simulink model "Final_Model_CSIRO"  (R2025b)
settings: Solver=ode23tb  StartTime=0.0  StopTime=50  RelTol=1e-3
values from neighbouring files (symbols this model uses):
  C_4 = 0.1670*C_b    (= 1.00487241952e-06)    [VSM_CSIRO.m]    (also in VSM.m)
  C_6 = 0.2835*C_b    (= 1.70587623314e-06)    [VSM_CSIRO.m]    (also in VSM.m)
  C_8 = 0.2275*C_b    (= 1.36891302659e-06)    [VSM_CSIRO.m]    (also in VSM.m)
  C_dc = 0.008*(n)    (= 1.6)    [VSM_CSIRO.m]    (also in VSM.m)
  C_f = n*300*10^-6    (= 0.06)    [VSM_CSIRO.m]    (also in VSM.m)
  D_p = (1/(m_p*w_b))    (= 101321.183642)    [VSM_CSIRO.m]    (also in VSM.m)
  droop_percentage = 1    [VSM_CSIRO.m]    (also in VSM.m = 5)
  i_ll = -1.15*(S_b/Vdc_n)-i_loss_dc    [VSM_CSIRO.m]    (also in VSM.m)
  i_ul = 1.15*(S_b/Vdc_n)+i_loss_dc    [VSM_CSIRO.m]    (also in VSM.m)
  J = D_p*tau_f    (= 2026.42367285)    [VSM_CSIRO.m]    (also in VSM.m)
  k_dc = eta_1/(Vdc_n*m_p)    [VSM_CSIRO.m]    (also in VSM.m)
  K_p = (1/Vdc_n)    [VSM_CSIRO.m]    (also in VSM.m)
  K_r = 1/R_dc    [VSM_CSIRO.m]    (also in VSM.m)
  Kff_i = 1    [VSM_CSIRO.m]    (also in VSM.m)
  Kff_v = 1    [VSM_CSIRO.m]    (also in VSM.m)
  Ki_i = (1/n)*1.19    (= 0.00595)    [VSM_CSIRO.m]    (also in VSM.m)
  Ki_v = (n)*1.161022    (= 232.2044)    [VSM_CSIRO.m]    (also in VSM.m)
  ki_v_ac = 4*5.2500e-04    (= 0.0021)    [VSM_CSIRO.m]    (also in VSM.m)
  Kp_i = 0.738891    [VSM_CSIRO.m]    (also in VSM.m)
  Kp_v = 0.52    [VSM_CSIRO.m]    (also in VSM.m)
  kp_v_ac = 0.001    [VSM_CSIRO.m]    (also in VSM.m)
  L1_pu = 1*0.0186/m    (= 0.000186)    [VSM_CSIRO.m]    (also in VSM.m)
  L_45 = L_lines(2)    [VSM_CSIRO.m]    (also in VSM.m)
  L_56 = L_lines(3)    [VSM_CSIRO.m]    (also in VSM.m)
  L_67 = L_lines(5)    [VSM_CSIRO.m]    (also in VSM.m)
  L_78 = L_lines(6)    [VSM_CSIRO.m]    (also in VSM.m)
  L_89 = L_lines(8)    [VSM_CSIRO.m]    (also in VSM.m)
  L_94 = L_lines(9)    [VSM_CSIRO.m]    (also in VSM.m)
  L_f = (1/n)*200*10^-6    (= 1e-06)    [VSM_CSIRO.m]    (also in VSM.m)
  n = 200    [VSM_CSIRO.m]    (also in VSM.m)
  pl = S_b*ps    (= 75000000)    [VSM_CSIRO.m]    (also in VSM.m)
  ps = base/3    (= 0.75)    [VSM_CSIRO.m]    (also in VSM.m)
  R1_pu = 1*0.00734/m    (= 7.34e-05)    [VSM_CSIRO.m]    (also in VSM.m)
  R_45 = R_lines(2)    [VSM_CSIRO.m]    (also in VSM.m)
  R_56 = R_lines(3)    [VSM_CSIRO.m]    (also in VSM.m)
  R_67 = R_lines(5)    [VSM_CSIRO.m]    (also in VSM.m)
  R_78 = R_lines(6)    [VSM_CSIRO.m]    (also in VSM.m)
  R_89 = R_lines(8)    [VSM_CSIRO.m]    (also in VSM.m)
  R_94 = R_lines(9)    [VSM_CSIRO.m]    (also in VSM.m)
  R_dc = (Vdc_n/(0.05*(S_b)/Vdc_n))    [VSM_CSIRO.m]    (also in VSM.m)
  R_f = 0.001/n    (= 5e-06)    [VSM_CSIRO.m]    (also in VSM.m)
  S_b = 100*(10^6)    (= 100000000)    [VSM_CSIRO.m]    (also in VSM.m)
  S_bt = S_b    (= 100000000)    [VSM_CSIRO.m]    (also in VSM.m)
  T_en = T_load-0.5    (= 44.5)    [VSM_CSIRO.m]    (also in VSM.m = 24.5)
  t_l = 2    [VSM_CSIRO.m]
  tau_dc = 0.05    [VSM_CSIRO.m]    (also in VSM.m)
  tau_g = 5    [VSM_CSIRO.m]    (also in VSM.m)
  V1_rms = 1000    [VSM_CSIRO.m]    (also in VSM.m)
  V2_rms = 13800    [VSM_CSIRO.m]    (also in VSM.m)
  V_m = sqrt(2/3)*V1_rms    [VSM_CSIRO.m]    (also in VSM.m)
  Vdc_n = 3*V_m    [VSM_CSIRO.m]    (also in VSM.m)
  w_b = 2*pi*f_b    (= 314.159265359)    [VSM_CSIRO.m]    (also in VSM.m)
  w_f = 2*pi*5    (= 31.4159265359)    [VSM_CSIRO.m]    (also in VSM.m)
undefined symbols (not defined in the file or in its folder): D1, Delta, DiscIntNeverNeededParam, i_dc
libraries: spsSeriesRLCBranchLib x142, spsThreePhaseVIMeasurementLib x69, slpidlib x44, spsabctodq0Lib x44, spsVoltageMeasurementLib x28, spsGroundLib x23, spsThreePhaseBreakerLib x23, spsThreePhaseParallelRLCLoadLib x21, spsdq0toabcLib x16, spsUniversalBridgeLib x16, spsPowerPositiveSequenceLib x14, spsDCVoltageSourceLib x14
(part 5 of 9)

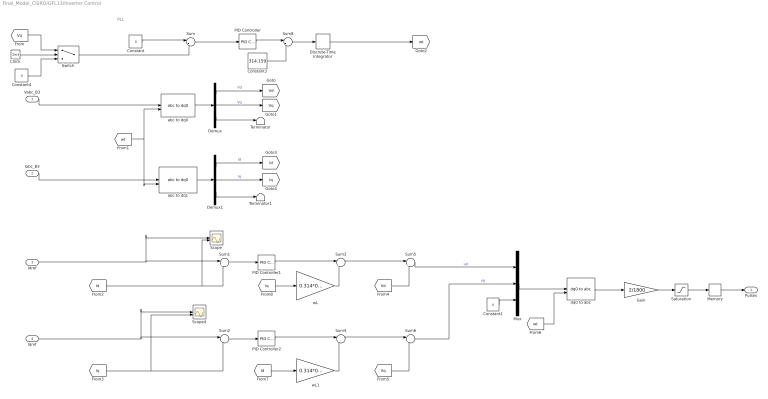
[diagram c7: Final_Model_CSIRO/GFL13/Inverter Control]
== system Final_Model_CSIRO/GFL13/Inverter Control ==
  note: PLL
  Vabc_B3 : Inport
  Iabc_B3 : Inport  Port=2
  Idref : Inport  Port=3
  Iqref : Inport  Port=4
  Clock : Clock
  Constant : Constant  Value=0  SampleTime=-1
  Constant1 : Constant  Value=0  SampleTime=-1
  Constant3 : Constant  Value=314.159  SampleTime=-1
  Constant4 : Constant  Value=0
  Demux : Demux  Outputs=3
  Demux1 : Demux  Outputs=3
  Discrete-Time Integrator : DiscreteIntegrator  SampleTime=-1  ICPrevOutput=DiscIntNeverNeededParam  ICPrevScaledInput=DiscIntNeverNeededParam
  Gain : Gain  Gain=2/1800
  Memory : Memory
  Mux : Mux  Inputs=3
  PID Controller : slpidlib/PID Controller  Controller=PI  Form=Parallel  TimeDomain=Discrete-time  UseExternalTs=off  SampleTime=-1  IntegratorMethod=Forward Euler  FilterMethod=Forward Euler  ControllerParametersSource=internal  P=0.02  I=50  UseKiTs=off  D=0  UseExternalDerivativeSource=off  N=100  UseFilter=on  TunerSelectOption=Transfer Function Based (PID Tuner App)  InitialConditionSource=internal  InitialConditionForIntegrator=0  InitialConditionForFilter=0  DifferentiatorICPrevScaledInput=0  ExternalReset=none  TrackingMode=off  Kt=1  LimitOutput=off  SatLimitsSource=internal  UpperSaturationLimit=inf  LowerSaturationLimit=-inf  LinearizeAsGain=on  AntiWindupMode=none  Kb=1  LimitIntegrator=off  UpperIntegratorSaturationLimit=inf  LowerIntegratorSaturationLimit=-inf  POutMin=[]  POutMax=[]  IOutMin=[]  IOutMax=[]  DOutMin=[]  DOutMax=[]  NOutMin=[]  NOutMax=[]  SumOutMin=[]  SumOutMax=[]  SaturationOutMin=[]  SaturationOutMax=[]  PParamMin=[]  PParamMax=[]  IParamMin=[]  IParamMax=[]  DParamMin=[]  DParamMax=[]  NParamMin=[]  NParamMax=[]  KbParamMin=[]  KbParamMax=[]  KtParamMin=[]  KtParamMax=[]  KbOutMin=[]  KbOutMax=[]  KtOutMin=[]  KtOutMax=[]  IntegratorOutMin=[]  IntegratorOutMax=[]  FilterOutMin=[]  FilterOutMax=[]  SumI1OutMin=[]  SumI1OutMax=[]  SumI2OutMin=[]  SumI2OutMax=[]  SumI3OutMin=[]  SumI3OutMax=[]  SumI4OutMin=[]  SumI4OutMax=[]  SumDOutMin=[]  SumDOutMax=[]  DifferentiatorOutMin=[]  DifferentiatorOutMax=[]  FilterDiffOutCoefMin=[]  FilterDiffOutCoefMax=[]  ReciprocalOutMin=[]  ReciprocalOutMax=[]  SumDenOutMin=[]  SumDenOutMax=[]  SumNumOutMin=[]  SumNumOutMax=[]  DivideOutMin=[]  DivideOutMax=[]  UdiffTsProdOutMin=[]  UdiffTsProdOutMax=[]  NTsProdOutMin=[]  NTsProdOutMax=[]  UintegralTsProdOutMin=[]  UintegralTsProdOutMax=[]  UngainTsProdOutMin=[]  UngainTsProdOutMax=[]  ClampingZeroOutDataTypeStr=Inherit: Inherit via back propagation  ClampingZeroOutMin=[]  ClampingZeroOutMax=[]  FilterDenConstantOutDataTypeStr=Inherit: Inherit via back propagation  FilterDenConstantOutMin=[]  FilterDenConstantOutMax=[]  PCopyOutDataTypeStr=Inherit: Inherit via back propagation  PCopyOutMin=[]  PCopyOutMax=[]  NCopyOutDataTypeStr=Inherit: Inherit via back propagation  NCopyOutMin=[]  NCopyOutMax=[]  IntegratorContinuousStateAttributes=''  IntegratorStateMustResolveToSignalObject=off  IntegratorRTWStateStorageClass=Auto  FilterContinuousStateAttributes=''  FilterStateMustResolveToSignalObject=off  FilterRTWStateStorageClass=Auto  ParallelPVariant=InternalParameters  IdealPVariant=Disabled  IVariant=InternalParameters  DVariant=Disabled  IntegratorVariant=Discrete  SatVariant=Disabled  AWVariant=Passthrough  PCopyVariant=Disabled  TRVariant=Disabled  FdbkBlocksVariant=Forward  IdealPFdbkVariant=Disabled  SatFdbkVariant=Disabled  DerivativeFilterVariant=Disabled  NVariant=Disabled  NCopyVariant=Disabled_SignalSpec  FilterICVariant=Disabled  IntegratorICVariant=InternalICs  ExternalResetVariant=Disabled  TRSumVariant=Passthrough  SumFdbkVariant=Disabled  SumVariant=Sum_PI  TsampFilterVariant=InternalTs  TsampNgainVariant=Passthrough  TsampIntegralVariant=Disabled_SignalSpec  ExternalSaturationOutDataTypeStr=Inherit: Same as second input  DerivativeSourceVariant=Disabled  PreIntVariant=InternalPreInt
  PID Controller1 : slpidlib/PID Controller  Controller=PI  Form=Parallel  TimeDomain=Discrete-time  UseExternalTs=off  SampleTime=-1  IntegratorMethod=Forward Euler  FilterMethod=Forward Euler  ControllerParametersSource=internal  P=0.1  I=10000/200  UseKiTs=off  D=0  UseExternalDerivativeSource=off  N=100  UseFilter=on  TunerSelectOption=Transfer Function Based (PID Tuner App)  InitialConditionSource=internal  InitialConditionForIntegrator=0  InitialConditionForFilter=0  DifferentiatorICPrevScaledInput=0  ExternalReset=none  TrackingMode=off  Kt=1  LimitOutput=on  SatLimitsSource=internal  UpperSaturationLimit=20e3  LowerSaturationLimit=-20e3  LinearizeAsGain=on  AntiWindupMode=none  Kb=1  LimitIntegrator=off  UpperIntegratorSaturationLimit=inf  LowerIntegratorSaturationLimit=-inf  POutMin=[]  POutMax=[]  IOutMin=[]  IOutMax=[]  DOutMin=[]  DOutMax=[]  NOutMin=[]  NOutMax=[]  SumOutMin=[]  SumOutMax=[]  SaturationOutMin=[]  SaturationOutMax=[]  PParamMin=[]  PParamMax=[]  IParamMin=[]  IParamMax=[]  DParamMin=[]  DParamMax=[]  NParamMin=[]  NParamMax=[]  KbParamMin=[]  KbParamMax=[]  KtParamMin=[]  KtParamMax=[]  KbOutMin=[]  KbOutMax=[]  KtOutMin=[]  KtOutMax=[]  IntegratorOutMin=[]  IntegratorOutMax=[]  FilterOutMin=[]  FilterOutMax=[]  SumI1OutMin=[]  SumI1OutMax=[]  SumI2OutMin=[]  SumI2OutMax=[]  SumI3OutMin=[]  SumI3OutMax=[]  SumI4OutMin=[]  SumI4OutMax=[]  SumDOutMin=[]  SumDOutMax=[]  DifferentiatorOutMin=[]  DifferentiatorOutMax=[]  FilterDiffOutCoefMin=[]  FilterDiffOutCoefMax=[]  ReciprocalOutMin=[]  ReciprocalOutMax=[]  SumDenOutMin=[]  SumDenOutMax=[]  SumNumOutMin=[]  SumNumOutMax=[]  DivideOutMin=[]  DivideOutMax=[]  UdiffTsProdOutMin=[]  UdiffTsProdOutMax=[]  NTsProdOutMin=[]  NTsProdOutMax=[]  UintegralTsProdOutMin=[]  UintegralTsProdOutMax=[]  UngainTsProdOutMin=[]  UngainTsProdOutMax=[]  ClampingZeroOutDataTypeStr=Inherit: Inherit via back propagation  ClampingZeroOutMin=[]  ClampingZeroOutMax=[]  FilterDenConstantOutDataTypeStr=Inherit: Inherit via back propagation  FilterDenConstantOutMin=[]  FilterDenConstantOutMax=[]  PCopyOutDataTypeStr=Inherit: Inherit via back propagation  PCopyOutMin=[]  PCopyOutMax=[]  NCopyOutDataTypeStr=Inherit: Inherit via back propagation  NCopyOutMin=[]  NCopyOutMax=[]  IntegratorContinuousStateAttributes=''  IntegratorStateMustResolveToSignalObject=off  IntegratorRTWStateStorageClass=Auto  FilterContinuousStateAttributes=''  FilterStateMustResolveToSignalObject=off  FilterRTWStateStorageClass=Auto  ParallelPVariant=InternalParameters  IdealPVariant=Disabled  IVariant=InternalParameters  DVariant=Disabled  IntegratorVariant=Discrete  SatVariant=Enabled  AWVariant=Passthrough  PCopyVariant=Disabled  TRVariant=Disabled  FdbkBlocksVariant=Forward  IdealPFdbkVariant=Disabled  SatFdbkVariant=Disabled  DerivativeFilterVariant=Disabled  NVariant=Disabled  NCopyVariant=Disabled_SignalSpec  FilterICVariant=Disabled  IntegratorICVariant=InternalICs  ExternalResetVariant=Disabled  TRSumVariant=Passthrough  SumFdbkVariant=Disabled  SumVariant=Sum_PI  TsampFilterVariant=InternalTs  TsampNgainVariant=Passthrough  TsampIntegralVariant=Disabled_SignalSpec  ExternalSaturationOutDataTypeStr=Inherit: Same as second input  DerivativeSourceVariant=Disabled  PreIntVariant=InternalPreInt
  PID Controller2 : slpidlib/PID Controller  Controller=PI  Form=Parallel  TimeDomain=Discrete-time  UseExternalTs=off  SampleTime=-1  IntegratorMethod=Forward Euler  FilterMethod=Forward Euler  ControllerParametersSource=internal  P=0.1  I=1000/2  UseKiTs=off  D=0  UseExternalDerivativeSource=off  N=100  UseFilter=on  TunerSelectOption=Transfer Function Based (PID Tuner App)  InitialConditionSource=internal  InitialConditionForIntegrator=0  InitialConditionForFilter=0  DifferentiatorICPrevScaledInput=0  ExternalReset=none  TrackingMode=off  Kt=1  LimitOutput=on  SatLimitsSource=internal  UpperSaturationLimit=20e3  LowerSaturationLimit=-20e3  LinearizeAsGain=on  AntiWindupMode=none  Kb=1  LimitIntegrator=off  UpperIntegratorSaturationLimit=inf  LowerIntegratorSaturationLimit=-inf  POutMin=[]  POutMax=[]  IOutMin=[]  IOutMax=[]  DOutMin=[]  DOutMax=[]  NOutMin=[]  NOutMax=[]  SumOutMin=[]  SumOutMax=[]  SaturationOutMin=[]  SaturationOutMax=[]  PParamMin=[]  PParamMax=[]  IParamMin=[]  IParamMax=[]  DParamMin=[]  DParamMax=[]  NParamMin=[]  NParamMax=[]  KbParamMin=[]  KbParamMax=[]  KtParamMin=[]  KtParamMax=[]  KbOutMin=[]  KbOutMax=[]  KtOutMin=[]  KtOutMax=[]  IntegratorOutMin=[]  IntegratorOutMax=[]  FilterOutMin=[]  FilterOutMax=[]  SumI1OutMin=[]  SumI1OutMax=[]  SumI2OutMin=[]  SumI2OutMax=[]  SumI3OutMin=[]  SumI3OutMax=[]  SumI4OutMin=[]  SumI4OutMax=[]  SumDOutMin=[]  SumDOutMax=[]  DifferentiatorOutMin=[]  DifferentiatorOutMax=[]  FilterDiffOutCoefMin=[]  FilterDiffOutCoefMax=[]  ReciprocalOutMin=[]  ReciprocalOutMax=[]  SumDenOutMin=[]  SumDenOutMax=[]  SumNumOutMin=[]  SumNumOutMax=[]  DivideOutMin=[]  DivideOutMax=[]  UdiffTsProdOutMin=[]  UdiffTsProdOutMax=[]  NTsProdOutMin=[]  NTsProdOutMax=[]  UintegralTsProdOutMin=[]  UintegralTsProdOutMax=[]  UngainTsProdOutMin=[]  UngainTsProdOutMax=[]  ClampingZeroOutDataTypeStr=Inherit: Inherit via back propagation  ClampingZeroOutMin=[]  ClampingZeroOutMax=[]  FilterDenConstantOutDataTypeStr=Inherit: Inherit via back propagation  FilterDenConstantOutMin=[]  FilterDenConstantOutMax=[]  PCopyOutDataTypeStr=Inherit: Inherit via back propagation  PCopyOutMin=[]  PCopyOutMax=[]  NCopyOutDataTypeStr=Inherit: Inherit via back propagation  NCopyOutMin=[]  NCopyOutMax=[]  IntegratorContinuousStateAttributes=''  IntegratorStateMustResolveToSignalObject=off  IntegratorRTWStateStorageClass=Auto  FilterContinuousStateAttributes=''  FilterStateMustResolveToSignalObject=off  FilterRTWStateStorageClass=Auto  ParallelPVariant=InternalParameters  IdealPVariant=Disabled  IVariant=InternalParameters  DVariant=Disabled  IntegratorVariant=Discrete  SatVariant=Enabled  AWVariant=Passthrough  PCopyVariant=Disabled  TRVariant=Disabled  FdbkBlocksVariant=Forward  IdealPFdbkVariant=Disabled  SatFdbkVariant=Disabled  DerivativeFilterVariant=Disabled  NVariant=Disabled  NCopyVariant=Disabled_SignalSpec  FilterICVariant=Disabled  IntegratorICVariant=InternalICs  ExternalResetVariant=Disabled  TRSumVariant=Passthrough  SumFdbkVariant=Disabled  SumVariant=Sum_PI  TsampFilterVariant=InternalTs  TsampNgainVariant=Passthrough  TsampIntegralVariant=Disabled_SignalSpec  ExternalSaturationOutDataTypeStr=Inherit: Same as second input  DerivativeSourceVariant=Disabled  PreIntVariant=InternalPreInt
  Saturation : Saturate  UpperLimit=1  LowerLimit=-1
  Scope : Scope  NumInputPorts=2
  Scope4 : Scope  NumInputPorts=2
  Sum : Sum  Inputs=|-+
  Sum1 : Sum  Inputs=|+-
  Sum2 : Sum  Inputs=|+-
  Sum3 : Sum  Inputs=|+-
  Sum{4..6,8} (4 alike) : Sum  Inputs=|++
  Switch : Switch  Criteria=u2 > Threshold  Threshold=10
  Terminator : Terminator
  Terminator1 : Terminator
  abc to dq0 : spsabctodq0Lib/abc to dq0  Alignment=90 degrees behind phase A axis
  abc to dq1 : spsabctodq0Lib/abc to dq0  Alignment=90 degrees behind phase A axis
  dq0 to abc : spsdq0toabcLib/dq0 to abc  Alignment=90 degrees behind phase A axis
  wL : Gain  Gain=0.314*0.003
  wL1 : Gain  Gain=0.314*0.003
  Pulses : Outport
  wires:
  abc to dq0/1 -> Demux/1
  Demux/3 -> Terminator/1
  Demux1/3 -> Terminator1/1
  abc to dq1/1 -> Demux1/1
  Iabc_B3/1 -> abc to dq1/1
  Constant/1 -> Sum/1
  Demux/2 -> [Vq]  "Vq"
  Sum/1 -> PID Controller/1
  PID Controller/1 -> Sum8/1
  [wt] -> abc to dq1/2, abc to dq0/2
  Demux1/1 -> [Id]  "Id"
  Demux1/2 -> [Iq]  "Iq"
  [Id] -> Scope/2, Sum1/2
  Iqref/1 -> Scope4/1, Sum2/1
  [Iq] -> Sum2/2, Scope4/2
  Sum1/1 -> PID Controller1/1
  Sum2/1 -> PID Controller2/1
  PID Controller1/1 -> Sum3/1
  PID Controller2/1 -> Sum4/1
  wL1/1 -> Sum4/2
  wL/1 -> Sum3/2
  Sum3/1 -> Sum5/1
  [Vd] -> Sum5/2
  Sum4/1 -> Sum6/1
  [Vq] -> Sum6/2
  Mux/1 -> dq0 to abc/1
  Sum5/1 -> Mux/1  "ud"
  Sum6/1 -> Mux/2  "uq"
  Constant1/1 -> Mux/3
  dq0 to abc/1 -> Gain/1
  Vabc_B3/1 -> abc to dq0/1
  Idref/1 -> Scope/1, Sum1/1
  [Id] -> wL1/1
  [Iq] -> wL/1
  Demux/1 -> [Vd]  "Vd"
  Gain/1 -> Saturation/1
  Memory/1 -> Pulses/1
  Discrete-Time Integrator/1 -> [wt]
  Saturation/1 -> Memory/1
  Constant3/1 -> Sum8/2
  Switch/1 -> Sum/2
  Constant4/1 -> Switch/3
  Clock/1 -> Switch/2
  [Vq] -> Switch/1
  [wt] -> dq0 to abc/2
  Sum8/1 -> Discrete-Time Integrator/1

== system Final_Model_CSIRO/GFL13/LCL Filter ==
  Cf : spsSeriesRLCBranchLib/Series RLC Branch  LConnTagsString=__new0  RConnTagsString=__new0  BranchType=RC  Resistance=200  Inductance=0.0058  SetiL0=off  InitialCurrent=0  Capacitance=50e-6  Setx0=off  InitialVoltage=0  Measurements=None
  Cf1 : spsSeriesRLCBranchLib/Series RLC Branch  LConnTagsString=__new0  RConnTagsString=__new0  BranchType=RC  Resistance=200  Inductance=0.0058  SetiL0=off  InitialCurrent=0  Capacitance=50e-6  Setx0=off  InitialVoltage=0  Measurements=None
  Cf2 : spsSeriesRLCBranchLib/Series RLC Branch  LConnTagsString=__new0  RConnTagsString=__new0  BranchType=RC  Resistance=200  Inductance=0.0058  SetiL0=off  InitialCurrent=0  Capacitance=50e-6  Setx0=off  InitialVoltage=0  Measurements=None
  Ground : spsGroundLib/Ground  LConnTagsString=a
  Lg : spsSeriesRLCBranchLib/Series RLC Branch  LConnTagsString=__new0  RConnTagsString=__new0  BranchType=L  Resistance=0.2  Inductance=5e-6  SetiL0=off  InitialCurrent=0  Capacitance=1e-6  Setx0=off  InitialVoltage=0  Measurements=None
  Linv : spsSeriesRLCBranchLib/Series RLC Branch  LConnTagsString=__new0  RConnTagsString=__new0  BranchType=RL  Resistance=1e-3  Inductance=0.003e-3  SetiL0=off  InitialCurrent=0  Capacitance=1e-6  Setx0=off  InitialVoltage=0  Measurements=None
  Series RLC Branch1 : spsSeriesRLCBranchLib/Series RLC Branch  LConnTagsString=__new0  RConnTagsString=__new0  BranchType=RL  Resistance=1e-3  Inductance=0.003e-3  SetiL0=off  InitialCurrent=0  Capacitance=1e-6  Setx0=off  InitialVoltage=0  Measurements=None
  Series RLC Branch2 : spsSeriesRLCBranchLib/Series RLC Branch  LConnTagsString=__new0  RConnTagsString=__new0  BranchType=RL  Resistance=1e-3  Inductance=0.003e-3  SetiL0=off  InitialCurrent=0  Capacitance=1e-6  Setx0=off  InitialVoltage=0  Measurements=None
  Series RLC Branch3 : spsSeriesRLCBranchLib/Series RLC Branch  LConnTagsString=__new0  RConnTagsString=__new0  BranchType=L  Resistance=0.2  Inductance=5e-6  SetiL0=off  InitialCurrent=0  Capacitance=1e-6  Setx0=off  InitialVoltage=0  Measurements=None
  Series RLC Branch4 : spsSeriesRLCBranchLib/Series RLC Branch  LConnTagsString=__new0  RConnTagsString=__new0  BranchType=L  Resistance=0.2  Inductance=5e-6  SetiL0=off  InitialCurrent=0  Capacitance=1e-6  Setx0=off  InitialVoltage=0  Measurements=None
  Three-Phase V-I Measurement : spsThreePhaseVIMeasurementLib/Three-Phase V-I Measurement  VoltageMeasurement=phase-to-phase  SetLabelV=on  LabelV=Vabc_B2_14  Vpu=off  VpuLL=off  CurrentMeasurement=no  SetLabelI=off  LabelI=Iabc  Ipu=off  Pbase=100e6  Vbase=500e3  OutputType=Complex  PhasorSimulation=off  PSBequivalent=0
  A : PMIOPort  Side=Left
  a : PMIOPort  Port=2  Side=Right
  B : PMIOPort  Port=3  Side=Left
  b : PMIOPort  Port=4  Side=Right
  C : PMIOPort  Port=5  Side=Left
  c : PMIOPort  Port=6  Side=Right
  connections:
  A/RConn1 -- Linv/LConn1
  B/RConn1 -- Series RLC Branch1/LConn1
  C/RConn1 -- Series RLC Branch2/LConn1
  Lg/LConn1 -- Three-Phase V-I Measurement/LConn1 -- Linv/RConn1
  Series RLC Branch4/LConn1 -- Three-Phase V-I Measurement/LConn3 -- Series RLC Branch2/RConn1
  Series RLC Branch3/LConn1 -- Three-Phase V-I Measurement/LConn2 -- Series RLC Branch1/RConn1
  Cf1/LConn1 -- Ground/LConn1 -- Cf/LConn1 -- Cf2/LConn1
  Cf/RConn1 -- Three-Phase V-I Measurement/RConn1
  Cf1/RConn1 -- Three-Phase V-I Measurement/RConn2
  Cf2/RConn1 -- Three-Phase V-I Measurement/RConn3
  Lg/RConn1 -- a/RConn1
  Series RLC Branch3/RConn1 -- b/RConn1
  Series RLC Branch4/RConn1 -- c/RConn1

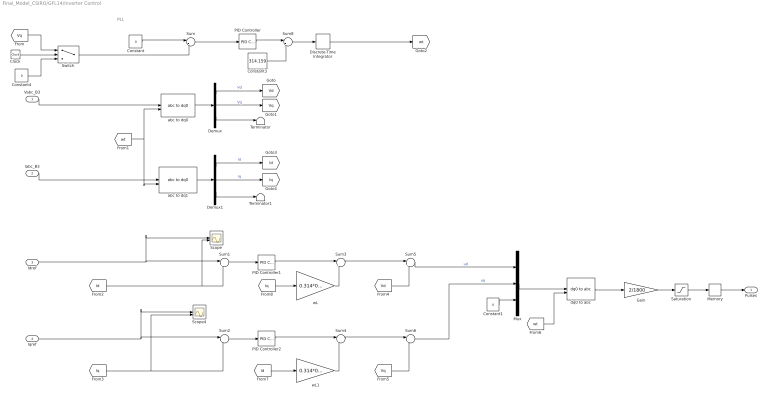
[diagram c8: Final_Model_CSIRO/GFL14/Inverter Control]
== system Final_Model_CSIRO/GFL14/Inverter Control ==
  note: PLL
  Vabc_B3 : Inport
  Iabc_B3 : Inport  Port=2
  Idref : Inport  Port=3
  Iqref : Inport  Port=4
  Clock : Clock
  Constant : Constant  Value=0  SampleTime=-1
  Constant1 : Constant  Value=0  SampleTime=-1
  Constant3 : Constant  Value=314.159  SampleTime=-1
  Constant4 : Constant  Value=0
  Demux : Demux  Outputs=3
  Demux1 : Demux  Outputs=3
  Discrete-Time Integrator : DiscreteIntegrator  SampleTime=-1  ICPrevOutput=DiscIntNeverNeededParam  ICPrevScaledInput=DiscIntNeverNeededParam
  Gain : Gain  Gain=2/1800
  Memory : Memory
  Mux : Mux  Inputs=3
  PID Controller : slpidlib/PID Controller  Controller=PI  Form=Parallel  TimeDomain=Discrete-time  UseExternalTs=off  SampleTime=-1  IntegratorMethod=Forward Euler  FilterMethod=Forward Euler  ControllerParametersSource=internal  P=0.02  I=50  UseKiTs=off  D=0  UseExternalDerivativeSource=off  N=100  UseFilter=on  TunerSelectOption=Transfer Function Based (PID Tuner App)  InitialConditionSource=internal  InitialConditionForIntegrator=0  InitialConditionForFilter=0  DifferentiatorICPrevScaledInput=0  ExternalReset=none  TrackingMode=off  Kt=1  LimitOutput=off  SatLimitsSource=internal  UpperSaturationLimit=inf  LowerSaturationLimit=-inf  LinearizeAsGain=on  AntiWindupMode=none  Kb=1  LimitIntegrator=off  UpperIntegratorSaturationLimit=inf  LowerIntegratorSaturationLimit=-inf  POutMin=[]  POutMax=[]  IOutMin=[]  IOutMax=[]  DOutMin=[]  DOutMax=[]  NOutMin=[]  NOutMax=[]  SumOutMin=[]  SumOutMax=[]  SaturationOutMin=[]  SaturationOutMax=[]  PParamMin=[]  PParamMax=[]  IParamMin=[]  IParamMax=[]  DParamMin=[]  DParamMax=[]  NParamMin=[]  NParamMax=[]  KbParamMin=[]  KbParamMax=[]  KtParamMin=[]  KtParamMax=[]  KbOutMin=[]  KbOutMax=[]  KtOutMin=[]  KtOutMax=[]  IntegratorOutMin=[]  IntegratorOutMax=[]  FilterOutMin=[]  FilterOutMax=[]  SumI1OutMin=[]  SumI1OutMax=[]  SumI2OutMin=[]  SumI2OutMax=[]  SumI3OutMin=[]  SumI3OutMax=[]  SumI4OutMin=[]  SumI4OutMax=[]  SumDOutMin=[]  SumDOutMax=[]  DifferentiatorOutMin=[]  DifferentiatorOutMax=[]  FilterDiffOutCoefMin=[]  FilterDiffOutCoefMax=[]  ReciprocalOutMin=[]  ReciprocalOutMax=[]  SumDenOutMin=[]  SumDenOutMax=[]  SumNumOutMin=[]  SumNumOutMax=[]  DivideOutMin=[]  DivideOutMax=[]  UdiffTsProdOutMin=[]  UdiffTsProdOutMax=[]  NTsProdOutMin=[]  NTsProdOutMax=[]  UintegralTsProdOutMin=[]  UintegralTsProdOutMax=[]  UngainTsProdOutMin=[]  UngainTsProdOutMax=[]  ClampingZeroOutDataTypeStr=Inherit: Inherit via back propagation  ClampingZeroOutMin=[]  ClampingZeroOutMax=[]  FilterDenConstantOutDataTypeStr=Inherit: Inherit via back propagation  FilterDenConstantOutMin=[]  FilterDenConstantOutMax=[]  PCopyOutDataTypeStr=Inherit: Inherit via back propagation  PCopyOutMin=[]  PCopyOutMax=[]  NCopyOutDataTypeStr=Inherit: Inherit via back propagation  NCopyOutMin=[]  NCopyOutMax=[]  IntegratorContinuousStateAttributes=''  IntegratorStateMustResolveToSignalObject=off  IntegratorRTWStateStorageClass=Auto  FilterContinuousStateAttributes=''  FilterStateMustResolveToSignalObject=off  FilterRTWStateStorageClass=Auto  ParallelPVariant=InternalParameters  IdealPVariant=Disabled  IVariant=InternalParameters  DVariant=Disabled  IntegratorVariant=Discrete  SatVariant=Disabled  AWVariant=Passthrough  PCopyVariant=Disabled  TRVariant=Disabled  FdbkBlocksVariant=Forward  IdealPFdbkVariant=Disabled  SatFdbkVariant=Disabled  DerivativeFilterVariant=Disabled  NVariant=Disabled  NCopyVariant=Disabled_SignalSpec  FilterICVariant=Disabled  IntegratorICVariant=InternalICs  ExternalResetVariant=Disabled  TRSumVariant=Passthrough  SumFdbkVariant=Disabled  SumVariant=Sum_PI  TsampFilterVariant=InternalTs  TsampNgainVariant=Passthrough  TsampIntegralVariant=Disabled_SignalSpec  ExternalSaturationOutDataTypeStr=Inherit: Same as second input  DerivativeSourceVariant=Disabled  PreIntVariant=InternalPreInt
  PID Controller1 : slpidlib/PID Controller  Controller=PI  Form=Parallel  TimeDomain=Discrete-time  UseExternalTs=off  SampleTime=-1  IntegratorMethod=Forward Euler  FilterMethod=Forward Euler  ControllerParametersSource=internal  P=0.1  I=10000/200  UseKiTs=off  D=0  UseExternalDerivativeSource=off  N=100  UseFilter=on  TunerSelectOption=Transfer Function Based (PID Tuner App)  InitialConditionSource=internal  InitialConditionForIntegrator=0  InitialConditionForFilter=0  DifferentiatorICPrevScaledInput=0  ExternalReset=none  TrackingMode=off  Kt=1  LimitOutput=on  SatLimitsSource=internal  UpperSaturationLimit=20e3  LowerSaturationLimit=-20e3  LinearizeAsGain=on  AntiWindupMode=none  Kb=1  LimitIntegrator=off  UpperIntegratorSaturationLimit=inf  LowerIntegratorSaturationLimit=-inf  POutMin=[]  POutMax=[]  IOutMin=[]  IOutMax=[]  DOutMin=[]  DOutMax=[]  NOutMin=[]  NOutMax=[]  SumOutMin=[]  SumOutMax=[]  SaturationOutMin=[]  SaturationOutMax=[]  PParamMin=[]  PParamMax=[]  IParamMin=[]  IParamMax=[]  DParamMin=[]  DParamMax=[]  NParamMin=[]  NParamMax=[]  KbParamMin=[]  KbParamMax=[]  KtParamMin=[]  KtParamMax=[]  KbOutMin=[]  KbOutMax=[]  KtOutMin=[]  KtOutMax=[]  IntegratorOutMin=[]  IntegratorOutMax=[]  FilterOutMin=[]  FilterOutMax=[]  SumI1OutMin=[]  SumI1OutMax=[]  SumI2OutMin=[]  SumI2OutMax=[]  SumI3OutMin=[]  SumI3OutMax=[]  SumI4OutMin=[]  SumI4OutMax=[]  SumDOutMin=[]  SumDOutMax=[]  DifferentiatorOutMin=[]  DifferentiatorOutMax=[]  FilterDiffOutCoefMin=[]  FilterDiffOutCoefMax=[]  ReciprocalOutMin=[]  ReciprocalOutMax=[]  SumDenOutMin=[]  SumDenOutMax=[]  SumNumOutMin=[]  SumNumOutMax=[]  DivideOutMin=[]  DivideOutMax=[]  UdiffTsProdOutMin=[]  UdiffTsProdOutMax=[]  NTsProdOutMin=[]  NTsProdOutMax=[]  UintegralTsProdOutMin=[]  UintegralTsProdOutMax=[]  UngainTsProdOutMin=[]  UngainTsProdOutMax=[]  ClampingZeroOutDataTypeStr=Inherit: Inherit via back propagation  ClampingZeroOutMin=[]  ClampingZeroOutMax=[]  FilterDenConstantOutDataTypeStr=Inherit: Inherit via back propagation  FilterDenConstantOutMin=[]  FilterDenConstantOutMax=[]  PCopyOutDataTypeStr=Inherit: Inherit via back propagation  PCopyOutMin=[]  PCopyOutMax=[]  NCopyOutDataTypeStr=Inherit: Inherit via back propagation  NCopyOutMin=[]  NCopyOutMax=[]  IntegratorContinuousStateAttributes=''  IntegratorStateMustResolveToSignalObject=off  IntegratorRTWStateStorageClass=Auto  FilterContinuousStateAttributes=''  FilterStateMustResolveToSignalObject=off  FilterRTWStateStorageClass=Auto  ParallelPVariant=InternalParameters  IdealPVariant=Disabled  IVariant=InternalParameters  DVariant=Disabled  IntegratorVariant=Discrete  SatVariant=Enabled  AWVariant=Passthrough  PCopyVariant=Disabled  TRVariant=Disabled  FdbkBlocksVariant=Forward  IdealPFdbkVariant=Disabled  SatFdbkVariant=Disabled  DerivativeFilterVariant=Disabled  NVariant=Disabled  NCopyVariant=Disabled_SignalSpec  FilterICVariant=Disabled  IntegratorICVariant=InternalICs  ExternalResetVariant=Disabled  TRSumVariant=Passthrough  SumFdbkVariant=Disabled  SumVariant=Sum_PI  TsampFilterVariant=InternalTs  TsampNgainVariant=Passthrough  TsampIntegralVariant=Disabled_SignalSpec  ExternalSaturationOutDataTypeStr=Inherit: Same as second input  DerivativeSourceVariant=Disabled  PreIntVariant=InternalPreInt
  PID Controller2 : slpidlib/PID Controller  Controller=PI  Form=Parallel  TimeDomain=Discrete-time  UseExternalTs=off  SampleTime=-1  IntegratorMethod=Forward Euler  FilterMethod=Forward Euler  ControllerParametersSource=internal  P=0.1  I=1000/2  UseKiTs=off  D=0  UseExternalDerivativeSource=off  N=100  UseFilter=on  TunerSelectOption=Transfer Function Based (PID Tuner App)  InitialConditionSource=internal  InitialConditionForIntegrator=0  InitialConditionForFilter=0  DifferentiatorICPrevScaledInput=0  ExternalReset=none  TrackingMode=off  Kt=1  LimitOutput=on  SatLimitsSource=internal  UpperSaturationLimit=20e3  LowerSaturationLimit=-20e3  LinearizeAsGain=on  AntiWindupMode=none  Kb=1  LimitIntegrator=off  UpperIntegratorSaturationLimit=inf  LowerIntegratorSaturationLimit=-inf  POutMin=[]  POutMax=[]  IOutMin=[]  IOutMax=[]  DOutMin=[]  DOutMax=[]  NOutMin=[]  NOutMax=[]  SumOutMin=[]  SumOutMax=[]  SaturationOutMin=[]  SaturationOutMax=[]  PParamMin=[]  PParamMax=[]  IParamMin=[]  IParamMax=[]  DParamMin=[]  DParamMax=[]  NParamMin=[]  NParamMax=[]  KbParamMin=[]  KbParamMax=[]  KtParamMin=[]  KtParamMax=[]  KbOutMin=[]  KbOutMax=[]  KtOutMin=[]  KtOutMax=[]  IntegratorOutMin=[]  IntegratorOutMax=[]  FilterOutMin=[]  FilterOutMax=[]  SumI1OutMin=[]  SumI1OutMax=[]  SumI2OutMin=[]  SumI2OutMax=[]  SumI3OutMin=[]  SumI3OutMax=[]  SumI4OutMin=[]  SumI4OutMax=[]  SumDOutMin=[]  SumDOutMax=[]  DifferentiatorOutMin=[]  DifferentiatorOutMax=[]  FilterDiffOutCoefMin=[]  FilterDiffOutCoefMax=[]  ReciprocalOutMin=[]  ReciprocalOutMax=[]  SumDenOutMin=[]  SumDenOutMax=[]  SumNumOutMin=[]  SumNumOutMax=[]  DivideOutMin=[]  DivideOutMax=[]  UdiffTsProdOutMin=[]  UdiffTsProdOutMax=[]  NTsProdOutMin=[]  NTsProdOutMax=[]  UintegralTsProdOutMin=[]  UintegralTsProdOutMax=[]  UngainTsProdOutMin=[]  UngainTsProdOutMax=[]  ClampingZeroOutDataTypeStr=Inherit: Inherit via back propagation  ClampingZeroOutMin=[]  ClampingZeroOutMax=[]  FilterDenConstantOutDataTypeStr=Inherit: Inherit via back propagation  FilterDenConstantOutMin=[]  FilterDenConstantOutMax=[]  PCopyOutDataTypeStr=Inherit: Inherit via back propagation  PCopyOutMin=[]  PCopyOutMax=[]  NCopyOutDataTypeStr=Inherit: Inherit via back propagation  NCopyOutMin=[]  NCopyOutMax=[]  IntegratorContinuousStateAttributes=''  IntegratorStateMustResolveToSignalObject=off  IntegratorRTWStateStorageClass=Auto  FilterContinuousStateAttributes=''  FilterStateMustResolveToSignalObject=off  FilterRTWStateStorageClass=Auto  ParallelPVariant=InternalParameters  IdealPVariant=Disabled  IVariant=InternalParameters  DVariant=Disabled  IntegratorVariant=Discrete  SatVariant=Enabled  AWVariant=Passthrough  PCopyVariant=Disabled  TRVariant=Disabled  FdbkBlocksVariant=Forward  IdealPFdbkVariant=Disabled  SatFdbkVariant=Disabled  DerivativeFilterVariant=Disabled  NVariant=Disabled  NCopyVariant=Disabled_SignalSpec  FilterICVariant=Disabled  IntegratorICVariant=InternalICs  ExternalResetVariant=Disabled  TRSumVariant=Passthrough  SumFdbkVariant=Disabled  SumVariant=Sum_PI  TsampFilterVariant=InternalTs  TsampNgainVariant=Passthrough  TsampIntegralVariant=Disabled_SignalSpec  ExternalSaturationOutDataTypeStr=Inherit: Same as second input  DerivativeSourceVariant=Disabled  PreIntVariant=InternalPreInt
  Saturation : Saturate  UpperLimit=1  LowerLimit=-1
  Scope : Scope  NumInputPorts=2
  Scope4 : Scope  NumInputPorts=2
  Sum : Sum  Inputs=|-+
  Sum1 : Sum  Inputs=|+-
  Sum2 : Sum  Inputs=|+-
  Sum3 : Sum  Inputs=|+-
  Sum{4..6,8} (4 alike) : Sum  Inputs=|++
  Switch : Switch  Criteria=u2 > Threshold  Threshold=10
  Terminator : Terminator
  Terminator1 : Terminator
  abc to dq0 : spsabctodq0Lib/abc to dq0  Alignment=90 degrees behind phase A axis
  abc to dq1 : spsabctodq0Lib/abc to dq0  Alignment=90 degrees behind phase A axis
  dq0 to abc : spsdq0toabcLib/dq0 to abc  Alignment=90 degrees behind phase A axis
  wL : Gain  Gain=0.314*0.003
  wL1 : Gain  Gain=0.314*0.003
  Pulses : Outport
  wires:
  abc to dq0/1 -> Demux/1
  Demux/3 -> Terminator/1
  Demux1/3 -> Terminator1/1
  abc to dq1/1 -> Demux1/1
  Iabc_B3/1 -> abc to dq1/1
  Constant/1 -> Sum/1
  Demux/2 -> [Vq]  "Vq"
  Sum/1 -> PID Controller/1
  PID Controller/1 -> Sum8/1
  [wt] -> abc to dq1/2, abc to dq0/2
  Demux1/1 -> [Id]  "Id"
  Demux1/2 -> [Iq]  "Iq"
  [Id] -> Scope/2, Sum1/2
  Iqref/1 -> Scope4/1, Sum2/1
  [Iq] -> Sum2/2, Scope4/2
  Sum1/1 -> PID Controller1/1
  Sum2/1 -> PID Controller2/1
  PID Controller1/1 -> Sum3/1
  PID Controller2/1 -> Sum4/1
  wL1/1 -> Sum4/2
  wL/1 -> Sum3/2
  Sum3/1 -> Sum5/1
  [Vd] -> Sum5/2
  Sum4/1 -> Sum6/1
  [Vq] -> Sum6/2
  Mux/1 -> dq0 to abc/1
  Sum5/1 -> Mux/1  "ud"
  Sum6/1 -> Mux/2  "uq"
  Constant1/1 -> Mux/3
  dq0 to abc/1 -> Gain/1
  Vabc_B3/1 -> abc to dq0/1
  Idref/1 -> Scope/1, Sum1/1
  [Id] -> wL1/1
  [Iq] -> wL/1
  Demux/1 -> [Vd]  "Vd"
  Gain/1 -> Saturation/1
  Memory/1 -> Pulses/1
  Discrete-Time Integrator/1 -> [wt]
  Saturation/1 -> Memory/1
  Constant3/1 -> Sum8/2
  Switch/1 -> Sum/2
  Constant4/1 -> Switch/3
  Clock/1 -> Switch/2
  [Vq] -> Switch/1
  [wt] -> dq0 to abc/2
  Sum8/1 -> Discrete-Time Integrator/1

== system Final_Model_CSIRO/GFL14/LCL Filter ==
  Cf : spsSeriesRLCBranchLib/Series RLC Branch  LConnTagsString=__new0  RConnTagsString=__new0  BranchType=RC  Resistance=200  Inductance=0.0058  SetiL0=off  InitialCurrent=0  Capacitance=50e-6  Setx0=off  InitialVoltage=0  Measurements=None
  Cf1 : spsSeriesRLCBranchLib/Series RLC Branch  LConnTagsString=__new0  RConnTagsString=__new0  BranchType=RC  Resistance=200  Inductance=0.0058  SetiL0=off  InitialCurrent=0  Capacitance=50e-6  Setx0=off  InitialVoltage=0  Measurements=None
  Cf2 : spsSeriesRLCBranchLib/Series RLC Branch  LConnTagsString=__new0  RConnTagsString=__new0  BranchType=RC  Resistance=200  Inductance=0.0058  SetiL0=off  InitialCurrent=0  Capacitance=50e-6  Setx0=off  InitialVoltage=0  Measurements=None
  Ground : spsGroundLib/Ground  LConnTagsString=a
  Lg : spsSeriesRLCBranchLib/Series RLC Branch  LConnTagsString=__new0  RConnTagsString=__new0  BranchType=L  Resistance=0.2  Inductance=5e-6  SetiL0=off  InitialCurrent=0  Capacitance=1e-6  Setx0=off  InitialVoltage=0  Measurements=None
  Linv : spsSeriesRLCBranchLib/Series RLC Branch  LConnTagsString=__new0  RConnTagsString=__new0  BranchType=RL  Resistance=1e-3  Inductance=0.003e-3  SetiL0=off  InitialCurrent=0  Capacitance=1e-6  Setx0=off  InitialVoltage=0  Measurements=None
  Series RLC Branch1 : spsSeriesRLCBranchLib/Series RLC Branch  LConnTagsString=__new0  RConnTagsString=__new0  BranchType=RL  Resistance=1e-3  Inductance=0.003e-3  SetiL0=off  InitialCurrent=0  Capacitance=1e-6  Setx0=off  InitialVoltage=0  Measurements=None
  Series RLC Branch2 : spsSeriesRLCBranchLib/Series RLC Branch  LConnTagsString=__new0  RConnTagsString=__new0  BranchType=RL  Resistance=1e-3  Inductance=0.003e-3  SetiL0=off  InitialCurrent=0  Capacitance=1e-6  Setx0=off  InitialVoltage=0  Measurements=None
  Series RLC Branch3 : spsSeriesRLCBranchLib/Series RLC Branch  LConnTagsString=__new0  RConnTagsString=__new0  BranchType=L  Resistance=0.2  Inductance=5e-6  SetiL0=off  InitialCurrent=0  Capacitance=1e-6  Setx0=off  InitialVoltage=0  Measurements=None
  Series RLC Branch4 : spsSeriesRLCBranchLib/Series RLC Branch  LConnTagsString=__new0  RConnTagsString=__new0  BranchType=L  Resistance=0.2  Inductance=5e-6  SetiL0=off  InitialCurrent=0  Capacitance=1e-6  Setx0=off  InitialVoltage=0  Measurements=None
  Three-Phase V-I Measurement : spsThreePhaseVIMeasurementLib/Three-Phase V-I Measurement  VoltageMeasurement=phase-to-phase  SetLabelV=on  LabelV=Vabc_B2_15  Vpu=off  VpuLL=off  CurrentMeasurement=no  SetLabelI=off  LabelI=Iabc  Ipu=off  Pbase=100e6  Vbase=500e3  OutputType=Complex  PhasorSimulation=off  PSBequivalent=0
  A : PMIOPort  Side=Left
  a : PMIOPort  Port=2  Side=Right
  B : PMIOPort  Port=3  Side=Left
  b : PMIOPort  Port=4  Side=Right
  C : PMIOPort  Port=5  Side=Left
  c : PMIOPort  Port=6  Side=Right
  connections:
  A/RConn1 -- Linv/LConn1
  B/RConn1 -- Series RLC Branch1/LConn1
  C/RConn1 -- Series RLC Branch2/LConn1
  Lg/LConn1 -- Three-Phase V-I Measurement/LConn1 -- Linv/RConn1
  Series RLC Branch4/LConn1 -- Three-Phase V-I Measurement/LConn3 -- Series RLC Branch2/RConn1
  Series RLC Branch3/LConn1 -- Three-Phase V-I Measurement/LConn2 -- Series RLC Branch1/RConn1
  Cf1/LConn1 -- Ground/LConn1 -- Cf/LConn1 -- Cf2/LConn1
  Cf/RConn1 -- Three-Phase V-I Measurement/RConn1
  Cf1/RConn1 -- Three-Phase V-I Measurement/RConn2
  Cf2/RConn1 -- Three-Phase V-I Measurement/RConn3
  Lg/RConn1 -- a/RConn1
  Series RLC Branch3/RConn1 -- b/RConn1
  Series RLC Branch4/RConn1 -- c/RConn1

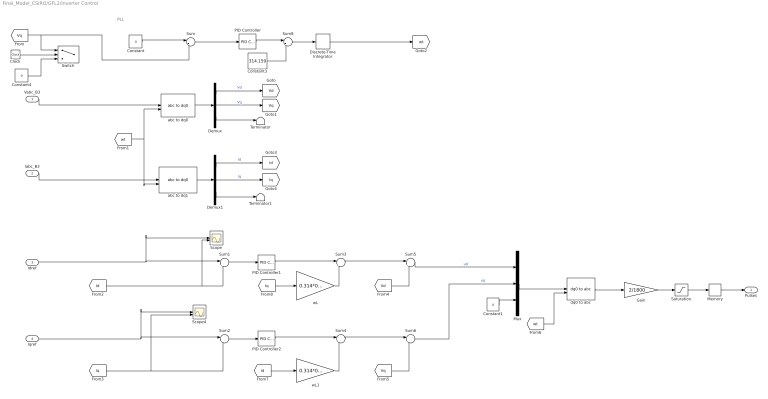
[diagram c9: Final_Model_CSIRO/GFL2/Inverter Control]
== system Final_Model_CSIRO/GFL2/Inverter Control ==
  note: PLL
  Vabc_B3 : Inport
  Iabc_B3 : Inport  Port=2
  Idref : Inport  Port=3
  Iqref : Inport  Port=4
  Clock : Clock
  Constant : Constant  Value=0  SampleTime=-1
  Constant1 : Constant  Value=0  SampleTime=-1
  Constant3 : Constant  Value=314.159  SampleTime=-1
  Constant4 : Constant  Value=0
  Demux : Demux  Outputs=3
  Demux1 : Demux  Outputs=3
  Discrete-Time Integrator : DiscreteIntegrator  SampleTime=-1  ICPrevOutput=DiscIntNeverNeededParam  ICPrevScaledInput=DiscIntNeverNeededParam
  Gain : Gain  Gain=2/1800
  Memory : Memory
  Mux : Mux  Inputs=3
  PID Controller : slpidlib/PID Controller  Controller=PI  Form=Parallel  TimeDomain=Discrete-time  UseExternalTs=off  SampleTime=-1  IntegratorMethod=Forward Euler  FilterMethod=Forward Euler  ControllerParametersSource=internal  P=0.02  I=50  UseKiTs=off  D=0  UseExternalDerivativeSource=off  N=100  UseFilter=on  TunerSelectOption=Transfer Function Based (PID Tuner App)  InitialConditionSource=internal  InitialConditionForIntegrator=0  InitialConditionForFilter=0  DifferentiatorICPrevScaledInput=0  ExternalReset=none  TrackingMode=off  Kt=1  LimitOutput=off  SatLimitsSource=internal  UpperSaturationLimit=inf  LowerSaturationLimit=-inf  LinearizeAsGain=on  AntiWindupMode=none  Kb=1  LimitIntegrator=off  UpperIntegratorSaturationLimit=inf  LowerIntegratorSaturationLimit=-inf  POutMin=[]  POutMax=[]  IOutMin=[]  IOutMax=[]  DOutMin=[]  DOutMax=[]  NOutMin=[]  NOutMax=[]  SumOutMin=[]  SumOutMax=[]  SaturationOutMin=[]  SaturationOutMax=[]  PParamMin=[]  PParamMax=[]  IParamMin=[]  IParamMax=[]  DParamMin=[]  DParamMax=[]  NParamMin=[]  NParamMax=[]  KbParamMin=[]  KbParamMax=[]  KtParamMin=[]  KtParamMax=[]  KbOutMin=[]  KbOutMax=[]  KtOutMin=[]  KtOutMax=[]  IntegratorOutMin=[]  IntegratorOutMax=[]  FilterOutMin=[]  FilterOutMax=[]  SumI1OutMin=[]  SumI1OutMax=[]  SumI2OutMin=[]  SumI2OutMax=[]  SumI3OutMin=[]  SumI3OutMax=[]  SumI4OutMin=[]  SumI4OutMax=[]  SumDOutMin=[]  SumDOutMax=[]  DifferentiatorOutMin=[]  DifferentiatorOutMax=[]  FilterDiffOutCoefMin=[]  FilterDiffOutCoefMax=[]  ReciprocalOutMin=[]  ReciprocalOutMax=[]  SumDenOutMin=[]  SumDenOutMax=[]  SumNumOutMin=[]  SumNumOutMax=[]  DivideOutMin=[]  DivideOutMax=[]  UdiffTsProdOutMin=[]  UdiffTsProdOutMax=[]  NTsProdOutMin=[]  NTsProdOutMax=[]  UintegralTsProdOutMin=[]  UintegralTsProdOutMax=[]  UngainTsProdOutMin=[]  UngainTsProdOutMax=[]  ClampingZeroOutDataTypeStr=Inherit: Inherit via back propagation  ClampingZeroOutMin=[]  ClampingZeroOutMax=[]  FilterDenConstantOutDataTypeStr=Inherit: Inherit via back propagation  FilterDenConstantOutMin=[]  FilterDenConstantOutMax=[]  PCopyOutDataTypeStr=Inherit: Inherit via back propagation  PCopyOutMin=[]  PCopyOutMax=[]  NCopyOutDataTypeStr=Inherit: Inherit via back propagation  NCopyOutMin=[]  NCopyOutMax=[]  IntegratorContinuousStateAttributes=''  IntegratorStateMustResolveToSignalObject=off  IntegratorRTWStateStorageClass=Auto  FilterContinuousStateAttributes=''  FilterStateMustResolveToSignalObject=off  FilterRTWStateStorageClass=Auto  ParallelPVariant=InternalParameters  IdealPVariant=Disabled  IVariant=InternalParameters  DVariant=Disabled  IntegratorVariant=Discrete  SatVariant=Disabled  AWVariant=Passthrough  PCopyVariant=Disabled  TRVariant=Disabled  FdbkBlocksVariant=Forward  IdealPFdbkVariant=Disabled  SatFdbkVariant=Disabled  DerivativeFilterVariant=Disabled  NVariant=Disabled  NCopyVariant=Disabled_SignalSpec  FilterICVariant=Disabled  IntegratorICVariant=InternalICs  ExternalResetVariant=Disabled  TRSumVariant=Passthrough  SumFdbkVariant=Disabled  SumVariant=Sum_PI  TsampFilterVariant=InternalTs  TsampNgainVariant=Passthrough  TsampIntegralVariant=Disabled_SignalSpec  ExternalSaturationOutDataTypeStr=Inherit: Same as second input  DerivativeSourceVariant=Disabled  PreIntVariant=InternalPreInt
  PID Controller1 : slpidlib/PID Controller  Controller=PI  Form=Parallel  TimeDomain=Discrete-time  UseExternalTs=off  SampleTime=-1  IntegratorMethod=Forward Euler  FilterMethod=Forward Euler  ControllerParametersSource=internal  P=0.1  I=10000/200  UseKiTs=off  D=0  UseExternalDerivativeSource=off  N=100  UseFilter=on  TunerSelectOption=Transfer Function Based (PID Tuner App)  InitialConditionSource=internal  InitialConditionForIntegrator=0  InitialConditionForFilter=0  DifferentiatorICPrevScaledInput=0  ExternalReset=none  TrackingMode=off  Kt=1  LimitOutput=on  SatLimitsSource=internal  UpperSaturationLimit=20e3  LowerSaturationLimit=-20e3  LinearizeAsGain=on  AntiWindupMode=none  Kb=1  LimitIntegrator=off  UpperIntegratorSaturationLimit=inf  LowerIntegratorSaturationLimit=-inf  POutMin=[]  POutMax=[]  IOutMin=[]  IOutMax=[]  DOutMin=[]  DOutMax=[]  NOutMin=[]  NOutMax=[]  SumOutMin=[]  SumOutMax=[]  SaturationOutMin=[]  SaturationOutMax=[]  PParamMin=[]  PParamMax=[]  IParamMin=[]  IParamMax=[]  DParamMin=[]  DParamMax=[]  NParamMin=[]  NParamMax=[]  KbParamMin=[]  KbParamMax=[]  KtParamMin=[]  KtParamMax=[]  KbOutMin=[]  KbOutMax=[]  KtOutMin=[]  KtOutMax=[]  IntegratorOutMin=[]  IntegratorOutMax=[]  FilterOutMin=[]  FilterOutMax=[]  SumI1OutMin=[]  SumI1OutMax=[]  SumI2OutMin=[]  SumI2OutMax=[]  SumI3OutMin=[]  SumI3OutMax=[]  SumI4OutMin=[]  SumI4OutMax=[]  SumDOutMin=[]  SumDOutMax=[]  DifferentiatorOutMin=[]  DifferentiatorOutMax=[]  FilterDiffOutCoefMin=[]  FilterDiffOutCoefMax=[]  ReciprocalOutMin=[]  ReciprocalOutMax=[]  SumDenOutMin=[]  SumDenOutMax=[]  SumNumOutMin=[]  SumNumOutMax=[]  DivideOutMin=[]  DivideOutMax=[]  UdiffTsProdOutMin=[]  UdiffTsProdOutMax=[]  NTsProdOutMin=[]  NTsProdOutMax=[]  UintegralTsProdOutMin=[]  UintegralTsProdOutMax=[]  UngainTsProdOutMin=[]  UngainTsProdOutMax=[]  ClampingZeroOutDataTypeStr=Inherit: Inherit via back propagation  ClampingZeroOutMin=[]  ClampingZeroOutMax=[]  FilterDenConstantOutDataTypeStr=Inherit: Inherit via back propagation  FilterDenConstantOutMin=[]  FilterDenConstantOutMax=[]  PCopyOutDataTypeStr=Inherit: Inherit via back propagation  PCopyOutMin=[]  PCopyOutMax=[]  NCopyOutDataTypeStr=Inherit: Inherit via back propagation  NCopyOutMin=[]  NCopyOutMax=[]  IntegratorContinuousStateAttributes=''  IntegratorStateMustResolveToSignalObject=off  IntegratorRTWStateStorageClass=Auto  FilterContinuousStateAttributes=''  FilterStateMustResolveToSignalObject=off  FilterRTWStateStorageClass=Auto  ParallelPVariant=InternalParameters  IdealPVariant=Disabled  IVariant=InternalParameters  DVariant=Disabled  IntegratorVariant=Discrete  SatVariant=Enabled  AWVariant=Passthrough  PCopyVariant=Disabled  TRVariant=Disabled  FdbkBlocksVariant=Forward  IdealPFdbkVariant=Disabled  SatFdbkVariant=Disabled  DerivativeFilterVariant=Disabled  NVariant=Disabled  NCopyVariant=Disabled_SignalSpec  FilterICVariant=Disabled  IntegratorICVariant=InternalICs  ExternalResetVariant=Disabled  TRSumVariant=Passthrough  SumFdbkVariant=Disabled  SumVariant=Sum_PI  TsampFilterVariant=InternalTs  TsampNgainVariant=Passthrough  TsampIntegralVariant=Disabled_SignalSpec  ExternalSaturationOutDataTypeStr=Inherit: Same as second input  DerivativeSourceVariant=Disabled  PreIntVariant=InternalPreInt
  PID Controller2 : slpidlib/PID Controller  Controller=PI  Form=Parallel  TimeDomain=Discrete-time  UseExternalTs=off  SampleTime=-1  IntegratorMethod=Forward Euler  FilterMethod=Forward Euler  ControllerParametersSource=internal  P=0.1  I=1000/2  UseKiTs=off  D=0  UseExternalDerivativeSource=off  N=100  UseFilter=on  TunerSelectOption=Transfer Function Based (PID Tuner App)  InitialConditionSource=internal  InitialConditionForIntegrator=0  InitialConditionForFilter=0  DifferentiatorICPrevScaledInput=0  ExternalReset=none  TrackingMode=off  Kt=1  LimitOutput=on  SatLimitsSource=internal  UpperSaturationLimit=20e3  LowerSaturationLimit=-20e3  LinearizeAsGain=on  AntiWindupMode=none  Kb=1  LimitIntegrator=off  UpperIntegratorSaturationLimit=inf  LowerIntegratorSaturationLimit=-inf  POutMin=[]  POutMax=[]  IOutMin=[]  IOutMax=[]  DOutMin=[]  DOutMax=[]  NOutMin=[]  NOutMax=[]  SumOutMin=[]  SumOutMax=[]  SaturationOutMin=[]  SaturationOutMax=[]  PParamMin=[]  PParamMax=[]  IParamMin=[]  IParamMax=[]  DParamMin=[]  DParamMax=[]  NParamMin=[]  NParamMax=[]  KbParamMin=[]  KbParamMax=[]  KtParamMin=[]  KtParamMax=[]  KbOutMin=[]  KbOutMax=[]  KtOutMin=[]  KtOutMax=[]  IntegratorOutMin=[]  IntegratorOutMax=[]  FilterOutMin=[]  FilterOutMax=[]  SumI1OutMin=[]  SumI1OutMax=[]  SumI2OutMin=[]  SumI2OutMax=[]  SumI3OutMin=[]  SumI3OutMax=[]  SumI4OutMin=[]  SumI4OutMax=[]  SumDOutMin=[]  SumDOutMax=[]  DifferentiatorOutMin=[]  DifferentiatorOutMax=[]  FilterDiffOutCoefMin=[]  FilterDiffOutCoefMax=[]  ReciprocalOutMin=[]  ReciprocalOutMax=[]  SumDenOutMin=[]  SumDenOutMax=[]  SumNumOutMin=[]  SumNumOutMax=[]  DivideOutMin=[]  DivideOutMax=[]  UdiffTsProdOutMin=[]  UdiffTsProdOutMax=[]  NTsProdOutMin=[]  NTsProdOutMax=[]  UintegralTsProdOutMin=[]  UintegralTsProdOutMax=[]  UngainTsProdOutMin=[]  UngainTsProdOutMax=[]  ClampingZeroOutDataTypeStr=Inherit: Inherit via back propagation  ClampingZeroOutMin=[]  ClampingZeroOutMax=[]  FilterDenConstantOutDataTypeStr=Inherit: Inherit via back propagation  FilterDenConstantOutMin=[]  FilterDenConstantOutMax=[]  PCopyOutDataTypeStr=Inherit: Inherit via back propagation  PCopyOutMin=[]  PCopyOutMax=[]  NCopyOutDataTypeStr=Inherit: Inherit via back propagation  NCopyOutMin=[]  NCopyOutMax=[]  IntegratorContinuousStateAttributes=''  IntegratorStateMustResolveToSignalObject=off  IntegratorRTWStateStorageClass=Auto  FilterContinuousStateAttributes=''  FilterStateMustResolveToSignalObject=off  FilterRTWStateStorageClass=Auto  ParallelPVariant=InternalParameters  IdealPVariant=Disabled  IVariant=InternalParameters  DVariant=Disabled  IntegratorVariant=Discrete  SatVariant=Enabled  AWVariant=Passthrough  PCopyVariant=Disabled  TRVariant=Disabled  FdbkBlocksVariant=Forward  IdealPFdbkVariant=Disabled  SatFdbkVariant=Disabled  DerivativeFilterVariant=Disabled  NVariant=Disabled  NCopyVariant=Disabled_SignalSpec  FilterICVariant=Disabled  IntegratorICVariant=InternalICs  ExternalResetVariant=Disabled  TRSumVariant=Passthrough  SumFdbkVariant=Disabled  SumVariant=Sum_PI  TsampFilterVariant=InternalTs  TsampNgainVariant=Passthrough  TsampIntegralVariant=Disabled_SignalSpec  ExternalSaturationOutDataTypeStr=Inherit: Same as second input  DerivativeSourceVariant=Disabled  PreIntVariant=InternalPreInt
  Saturation : Saturate  UpperLimit=1  LowerLimit=-1
  Scope : Scope  NumInputPorts=2
  Scope4 : Scope  NumInputPorts=2
  Sum : Sum  Inputs=|-+
  Sum1 : Sum  Inputs=|+-
  Sum2 : Sum  Inputs=|+-
  Sum3 : Sum  Inputs=|+-
  Sum{4..6,8} (4 alike) : Sum  Inputs=|++
  Switch : Switch  Criteria=u2 > Threshold  Threshold=10
  Terminator : Terminator
  Terminator1 : Terminator
  abc to dq0 : spsabctodq0Lib/abc to dq0  Alignment=90 degrees behind phase A axis
  abc to dq1 : spsabctodq0Lib/abc to dq0  Alignment=90 degrees behind phase A axis
  dq0 to abc : spsdq0toabcLib/dq0 to abc  Alignment=90 degrees behind phase A axis
  wL : Gain  Gain=0.314*0.003
  wL1 : Gain  Gain=0.314*0.003
  Pulses : Outport
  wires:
  abc to dq0/1 -> Demux/1
  Demux/3 -> Terminator/1
  Demux1/3 -> Terminator1/1
  abc to dq1/1 -> Demux1/1
  Iabc_B3/1 -> abc to dq1/1
  Constant/1 -> Sum/1
  Demux/2 -> [Vq]  "Vq"
  Sum/1 -> PID Controller/1
  PID Controller/1 -> Sum8/1
  [wt] -> abc to dq1/2, abc to dq0/2
  Demux1/1 -> [Id]  "Id"
  Demux1/2 -> [Iq]  "Iq"
  [Id] -> Scope/2, Sum1/2
  Iqref/1 -> Scope4/1, Sum2/1
  [Iq] -> Sum2/2, Scope4/2
  Sum1/1 -> PID Controller1/1
  Sum2/1 -> PID Controller2/1
  PID Controller1/1 -> Sum3/1
  PID Controller2/1 -> Sum4/1
  wL1/1 -> Sum4/2
  wL/1 -> Sum3/2
  Sum3/1 -> Sum5/1
  [Vd] -> Sum5/2
  Sum4/1 -> Sum6/1
  [Vq] -> Sum6/2
  Mux/1 -> dq0 to abc/1
  Sum5/1 -> Mux/1  "ud"
  Sum6/1 -> Mux/2  "uq"
  Constant1/1 -> Mux/3
  dq0 to abc/1 -> Gain/1
  Vabc_B3/1 -> abc to dq0/1
  Idref/1 -> Scope/1, Sum1/1
  [Id] -> wL1/1
  [Iq] -> wL/1
  Demux/1 -> [Vd]  "Vd"
  Gain/1 -> Saturation/1
  Memory/1 -> Pulses/1
  Discrete-Time Integrator/1 -> [wt]
  Saturation/1 -> Memory/1
  Constant3/1 -> Sum8/2
  Constant4/1 -> Switch/3
  Clock/1 -> Switch/2
  [Vq] -> Sum/2, Switch/1
  [wt] -> dq0 to abc/2
  Sum8/1 -> Discrete-Time Integrator/1
